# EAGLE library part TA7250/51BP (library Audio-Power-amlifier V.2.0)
30W BTL Audio Power Amplifier of Toshiba Bipolar Linear.
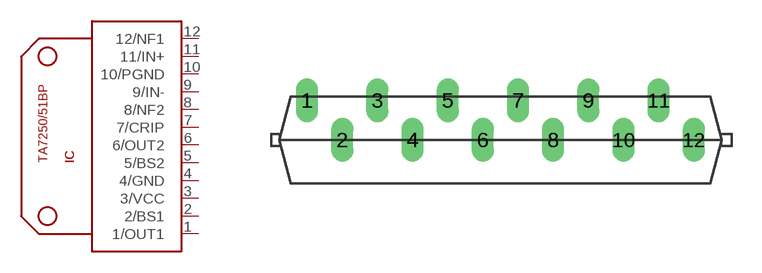
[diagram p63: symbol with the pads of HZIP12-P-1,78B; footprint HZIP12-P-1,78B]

Designator prefix IC

## TA7250/51BP  [HZIP12-P-1,78B]
1  1/OUT1  out
2  2/BS1
3  3/VCC  pwr
4  4/GND  pwr
5  5/BS2
6  6/OUT2  out
7  7/CRIP
8  8/NF2
9  9/IN-  in
10  10/PGND  pwr
11  11/IN+  in
12  12/NF1

## Footprint HZIP12-P-1,78B (pad centres in mm)
drill 0.6 pad 1.016 long: 1 -9.779,2; 2 -8.001,0; 3 -6.223,2; 4 -4.445,0; 5 -2.667,2; 6 -0.889,0; 7 0.889,2; 8 2.667,0; 9 4.445,2; 10 6.223,0; 11 8.001,2; 12 9.779,0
